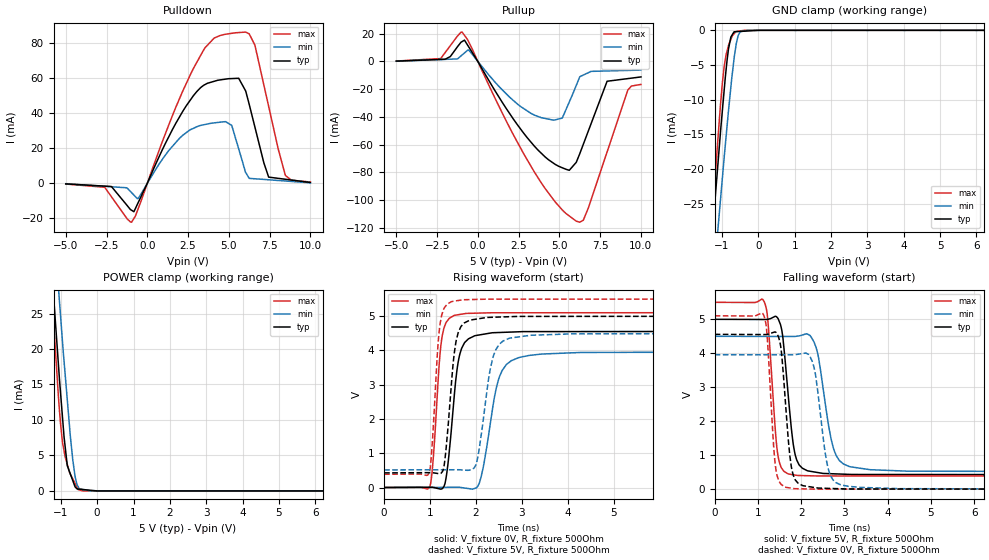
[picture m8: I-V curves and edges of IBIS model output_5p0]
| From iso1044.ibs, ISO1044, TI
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|   output_5p0 Model
[Model]   output_5p0
Model_type   3-state
Polarity   Inverting
Vmeas = 2.5
Vref = 0
Cref = 2pF
Rref = 100000
|   typ   min   max
C_comp   1.147pF   1.101pF   1.224pF
|C_comp_pullup   1.018pF   1.046pF   1.061pF
|C_comp_pulldown   0.963pF   0.985pF   1.013pF
|  Where Nom  PVT is Nominal Process, 5.0V,   27C
|   Fast PVT is Strong Process,  4.5V,   -40C
|   Slow PVT is Weak Process,   5.5V,   150C
[Voltage Range]   5   4.5   5.5
|Junction Temperature
[Temperature Range]   27   150   -40
[Pullup Reference]   5   4.5   5.5
[Pulldown Reference]   -0   -0   0
[Power Clamp Reference]   5   4.5   5.5
[GND Clamp Reference]   0   0   0
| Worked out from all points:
|   slope of the pulldown table from 0 to 0.75 V, typ, clamps not added: 47.7 ohm
|   slope of the pullup table from 0 to 0.75 V, typ, clamps not added: 49.3 ohm
|   GND clamp passes 1 mA (typ) near -0.76 V on its own axis
|   POWER clamp passes 1 mA (typ) near -0.64 V on its own axis
|   falling waveform, V_fixture 5V, R_fixture 500Ohm: 20-80 % time 209ps typ, 302ps min, 165ps max; typ from 5 V to 0.427 V
|   rising waveform, V_fixture 0V, R_fixture 500Ohm: 20-80 % time 202ps typ, 310ps min, 152ps max; typ from 0 V to 4.56 V
|   rising waveform, V_fixture 5V, R_fixture 500Ohm: 20-80 % time 183ps typ, 263ps min, 139ps max; typ from 0.427 V to 5 V
|   falling waveform, V_fixture 0V, R_fixture 500Ohm: 20-80 % time 175ps typ, 240ps min, 143ps max; typ from 4.56 V to 0 V
[Pulldown]
|   Voltage   I(typ)   I(min)   I(max)
-5V       -326.8uA   -210.4uA   -409.2uA
-2.61V    -1.601mA   -1.7mA     -2.259mA
-962.9mV  -15.39mA   -5.332mA   -22.21mA
-529.2mV  -10.45mA   -8.292mA   -13.78mA
2.178V    41.19mA    27.48mA    52.8mA
3.892V    57.73mA    34.3mA     80.94mA
5.177V    59.86mA    33.12mA    85.72mA
6.034V    52.75mA    6.206mA    86.43mA
6.601V    32.08mA    2.603mA    78.91mA
7.442V    3.552mA    2.03mA     44.02mA
8.467V    2.319mA    1.332mA    4.54mA
10V       476.2uA    287.2uA    755.3uA
[GND Clamp]
|   Voltage   I(typ)   I(min)   I(max)
-5V       -292.8mA   -279.1mA   -331.6mA
-1.43V    -40.73mA   -48.41mA   -40.04mA
-1.25V    -28.34mA   -37.04mA   -25.96mA
-1.138V   -21.05mA   -30.32mA   -17.59mA
-1.054V   -15.57mA   -25.26mA   -11.67mA
-940.9mV  -8.727mA   -18.42mA   -5.257mA
-821.2mV  -2.708mA   -11.63mA   -2.234mA
-754.9mV  -961.8uA   -8.181mA   -1.305mA
-666.4mV  -212uA     -4.028mA   -482uA
-555.1mV  -176.6uA   -757.5uA   -128.1uA
-298.6mV  -94.99uA   -1.118uA   -331.7nA
10V       0A         0A         0A
[Pullup]
|   Voltage   I(typ)   I(min)   I(max)
-5V       272.2uA    178.9uA    326.4uA
-2.281V   1.495mA    1.403mA    2.101mA
-966.2mV  14.38mA    4.716mA    21.22mA
-558.9mV  10.48mA    8.11mA     14.11mA
2.41V     -45.41mA   -30.55mA   -57.94mA
4.535V    -72.55mA   -42.08mA   -98.09mA
5.176V    -76.69mA   -40.83mA   -107.1mA
5.606V    -78.52mA   -29.22mA   -111.5mA
6.25V     -66.5mA    -10.99mA   -116mA
7.925V    -14.26mA   -6.833mA   -65.3mA
9.195V    -12.35mA   -6.448mA   -20.62mA
10V       -11.14mA   -6.205mA   -16.55mA
[POWER Clamp]
|   Voltage   I(typ)   I(min)   I(max)
-5V       414.2mA    345.9mA    503.1mA
-1.25V    31.21mA    41.3mA     27.86mA
-1.062V   17.59mA    28.48mA    13.08mA
-1.036V   15.65mA    26.65mA    11.25mA
-952.9mV  10.35mA    20.99mA    6.844mA
-910mV    7.594mA    18.25mA    5.634mA
-821.5mV  3.556mA    12.83mA    3.74mA
-670.3mV  1.45mA     4.372mA    1.687mA
-607.2mV  570.5uA    2.045mA    1.049mA
-521.8mV  263.4uA    587.9uA    185.7uA
-178.8mV  90.21uA    340.1nA    3.201uA
10V       0A         0A         0A
[Ramp]
R_load = 500
|   typ   min   max
dV/dt_r   2.73397/2.0226e-10   2.37519/3.08766e-10   3.06172/1.51533e-10
dV/dt_f   2.74387/2.0786e-10   2.3921/2.99656e-10   3.06824/1.65021e-10
[Falling Waveform]
V_fixture = 5V
V_fixture_min = 4.5V
V_fixture_max = 5.5V
R_fixture = 500Ohm
C_fixture = 0F
|   Time   V(typ)   V(min)   V(max)
0s        5V         4.5V       5.5V
1.149ns   4.995V     4.497V     5.51V
1.229ns   5V         4.496V     4.978V
1.449ns   5.049V     4.496V     1.114V
1.69ns    2.917V     4.495V     455.4mV
1.957ns   707.4mV    4.513V     401.9mV
2.304ns   506.1mV    4.312V     390.9mV
2.742ns   452.2mV    1.227V     388.4mV
3.112ns   435.3mV    667.4mV    388.3mV
10ns      426.9mV    513.1mV    386.3mV
[Rising Waveform]
V_fixture = 0V
V_fixture_min = 0V
V_fixture_max = 0V
R_fixture = 500Ohm
C_fixture = 0F
|   Time   V(typ)   V(min)   V(max)
0s        -120.9nV   96.02uV    1.534nV
995.7ps   6.33mV     3.678mV    28.2mV
1.254ns   -39.67mV   4.609mV    4.323V
1.368ns   438mV      5.017mV    4.847V
1.52ns    2.542V     5.565mV    5.018V
1.689ns   4.06V      -2.475mV   5.059V
2.045ns   4.446V     44.29mV    5.09V
2.495ns   4.524V     3.156V     5.1V
2.932ns   4.545V     3.79V      5.1V
10ns      4.557V     3.959V     5.103V
[Rising Waveform]
V_fixture = 5V
V_fixture_min = 4.5V
V_fixture_max = 5.5V
R_fixture = 500Ohm
C_fixture = 0F
|   Time   V(typ)   V(min)   V(max)
0s        426.9mV    513.1mV    386.3mV
979.2ps   433.3mV    516.4mV    420.4mV
1.215ns   403.1mV    517.2mV    4.725V
1.322ns   782.7mV    517.5mV    5.263V
1.464ns   2.972V     518mV      5.422V
1.612ns   4.509V     518.5mV    5.458V
1.994ns   4.912V     648.3mV    5.489V
2.364ns   4.969V     3.756V     5.497V
2.722ns   4.985V     4.353V     5.498V
10ns      5V         4.5V       5.5V
[Falling Waveform]
|Gnd
V_fixture = 0V
V_fixture_min = 0V
V_fixture_max = 0V
R_fixture = 500Ohm
C_fixture = 0F
|   Time   V(typ)   V(min)   V(max)
0s        4.557V     3.959V     5.103V
1.133ns   4.551V     3.956V     5.125V
1.209ns   4.552V     3.955V     4.576V
1.406ns   4.623V     3.955V     670.5mV
1.63ns    2.663V     3.954V     62.26mV
1.867ns   266mV      3.96V      14.27mV
2.265ns   57.53mV    3.731V     2.216mV
2.622ns   23.57mV    622.2mV    1.666mV
2.912ns   11.72mV    130.1mV    1.6mV
10ns      -38.64nV   96.1uV     -33.33nV
